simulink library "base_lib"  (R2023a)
settings: Solver=VariableStepAuto  StartTime=0.0  StopTime=10.0  RelTol=1e-3
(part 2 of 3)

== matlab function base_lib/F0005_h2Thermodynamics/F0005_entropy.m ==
function s = F0005_entropy(T,rho)
%ENTROPY
%    S = ENTROPY(T,RHO)

%    This function was generated by the Symbolic Math Toolbox version 8.7.
%    04-Nov-2021 19:06:03

t2 = rho.^2;
t3 = rho.^3;
t5 = 1.0./T;
t6 = rho./1.5508e+4;
t4 = t2.^2;
t7 = -t6;
t9 = t5.*3.3145e+1;
t10 = t6-3.9e+1./2.5e+2;
t11 = t6-6.7e+1./1.0e+2;
t12 = t6-2.17e+2./1.25e+2;
t13 = t6-7.53e+2./5.0e+2;
t14 = t6-8.31e+2./5.0e+2;
t55 = t5.*6.858999999999336e+3;
t56 = t5.*5.309999999993605e+2;
t57 = t5.*1.98899999999884e+3;
t59 = t5.*2.484000000001446e+3;
t60 = t5.*7.51000000000887e+2;
t8 = exp(t7);
t15 = t10.^2;
t16 = t11.^2;
t17 = t12.^2;
t18 = t13.^2;
t19 = t14.^2;
t20 = t9.^2.986;
t21 = t9.^5.646;
t22 = t9.^(7.91e+2./1.0e+3);
t23 = t9.^4.187;
t24 = t9.^7.249;
t25 = t9-7.164e-1;
t26 = t9-7.204e-1;
t27 = t9-1.5445;
t28 = t9-1.3444;
t29 = t9-1.4517;
t58 = -t55;
t61 = -t56;
t62 = -t57;
t63 = -t59;
t64 = -t60;
t30 = t25.^2;
t31 = t26.^2;
t32 = t27.^2;
t33 = t28.^2;
t34 = t29.^2;
t35 = t15.*(4.89e+2./1.0e+3);
t36 = t17.*(1.03e+2./1.0e+3);
t38 = t18.*(3.37e+2./2.0e+2);
t39 = t16.*2.506;
t43 = t19.*1.607;
t65 = exp(t58);
t66 = exp(t61);
t67 = exp(t62);
t68 = exp(t63);
t69 = exp(t64);
t37 = -t35;
t40 = -t36;
t41 = -t38;
t42 = -t39;
t44 = -t43;
t45 = t30.*(1.71e+2./1.0e+3);
t46 = t33.*2.245e-1;
t48 = t31.*2.785e-1;
t51 = t32.*3.967e-1;
t52 = t34.*1.304e-1;
t47 = -t45;
t49 = -t46;
t50 = -t48;
t53 = -t51;
t54 = -t52;
t70 = t37+t49;
t71 = t41+t47;
t73 = t42+t50;
t75 = t40+t54;
t78 = t44+t53;
t72 = exp(t70);
t74 = exp(t71);
t76 = exp(t73);
t77 = exp(t75);
t79 = exp(t78);
et1 = T.*4.525569467491326e-2+t4./5.78393187877481e+18-(t65.*2.518450143309456e+2)./(t65-1.0)-(t66.*2.58891537184784e+1)./(t66-1.0)+(t67.*4.75271685020088e+1)./(t67-1.0);
et2 = (t68.*(-5.68071202293286e+1))./(t68-1.0)+(t69.*9.32830592850702)./(t69-1.0)+rho.*1.0./t9.^(1.1e+1./1.0e+3).*1.345685388186742e-4+rho.*1.0./t9.^(5.11e+2./1.0e+3).*1.425437522568997e-4;
et3 = rho.*1.0./t9.^3.156e-1.*(-3.061189509930358e-4)+t2.*1.0./t9.^(1.97e+2./1.0e+3).*2.445961028609361e-9+t3.*t9.^(4.09e+2./1.0e+3).*4.94840435608013e-14;
et4 = t2.*t9.^1.444e-1.*(-6.380426347215835e-9)-rho.*t8.*t9.^(3.77e+2./5.0e+2).*8.792778927005417e-5+rho.*t9.^(9.93e+2./5.0e+2).*t79.*1.073146218725819e-5;
et5 = rho.*t9.^4.646.*t72.*8.239344544751096e-6-rho.*t9.^6.249.*t76.*1.083292654114006e-5+t3.*1.0./t9.^(2.09e+2./1.0e+3).*t77.*6.826366580922388e-15;
et6 = t3.*t8.*t9.^(3.11e+2./1.0e+3).*1.237111603428444e-13-t2.*t9.^3.187.*t74.*3.685912798034e-10;
et7 = rho.*t21.*t72.*(t5.*1.4882105e+1-6.036356e-1).*(-1.459324219757545e-6)+rho.*t24.*t76.*(t5.*1.8461765e+1-4.012628e-1).*1.494402888831571e-6;
et8 = t2.*t23.*t74.*(t5.*1.133559e+1-2.450088e-1).*8.803230948254119e-11-t3.*t22.*t77.*(t5.*8.644216-3.7860336e-1).*8.630046246425269e-15;
et9 = rho.*t20.*t79.*(t5.*2.6297243e+1-1.2254063).*(-3.593925715759608e-6)+1.888076782;
et10 = t5.*(-5.203221931700199e+2)-log(-t65+1.0).*1.0118712424e+1-log(-t66+1.0).*1.3436186752e+1;
et11 = log(-t67+1.0).*6.585061824-log(-t68+1.0).*6.302369776+log(-t69+1.0).*3.4230681224-log(t6).*8.314472;
et12 = log(t9).*(-1.2471708e+1)-t4.*t5.*4.764633820313524e-17-rho.*t9.^(4.89e+2./1.0e+3).*2.423672877126645e-3;
et13 = rho.*t9.^(9.89e+2./1.0e+3).*(-1.131310766520506e-3)+rho.*t9.^6.844e-1.*3.718903341176167e-3;
et14 = t2.*t9.^(8.03e+2./1.0e+3).*(-2.532612015624375e-8)-t3.*t9.^1.409.*2.920040416132454e-13;
et15 = t2.*t9.^1.1444.*4.635606100313556e-8+t5.*(et1+et2+et3+et4+et5+et6+et7+et8+et9).*2.7558317444e+2+rho.*t8.*t9.^(8.77e+2./5.0e+2).*4.168033876327057e-4;
et16 = t3.*t8.*t9.^1.311.*(-7.845865589306564e-13)-rho.*t21.*t72.*1.213351036409595e-5;
et17 = rho.*t20.*t79.*(-2.988159473376322e-5)+rho.*t24.*t76.*1.242517097590921e-5;
et18 = t2.*t23.*t74.*7.319421722879233e-10-t3.*t22.*t77.*7.1754277874608e-14;
et19 = 1.212238084254062e+1;
s = et10+et11+et12+et13+et14+et15+et16+et17+et18+et19;

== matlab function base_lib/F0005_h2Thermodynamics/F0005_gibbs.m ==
function g = F0005_gibbs(T,rho)
%GIBBSENERGY
%    G = GIBBSENERGY(T,RHO)

%    This function was generated by the Symbolic Math Toolbox version 8.7.
%    04-Nov-2021 19:06:06

t2 = rho.^2;
t3 = rho.^3;
t4 = 1.0./T;
t5 = rho./1.5508e+4;
t6 = -t5;
t8 = t4.*3.3145e+1;
t9 = t5-3.9e+1./2.5e+2;
t10 = t5-6.7e+1./1.0e+2;
t11 = t5-2.17e+2./1.25e+2;
t12 = t5-7.53e+2./5.0e+2;
t13 = t5-8.31e+2./5.0e+2;
t7 = exp(t6);
t14 = t9.^2;
t15 = t10.^2;
t16 = t11.^2;
t17 = t12.^2;
t18 = t13.^2;
t19 = t8.^(8.77e+2./5.0e+2);
t20 = t8.^(4.89e+2./1.0e+3);
t21 = t8.^2.986;
t22 = t8.^5.646;
t23 = t8.^(7.91e+2./1.0e+3);
t24 = t8.^(8.03e+2./1.0e+3);
t25 = t8.^(9.89e+2./1.0e+3);
t26 = t8.^1.311;
t27 = t8.^1.409;
t28 = t8.^6.844e-1;
t29 = t8.^4.187;
t30 = t8.^1.1444;
t31 = t8.^7.249;
t32 = t8-7.164e-1;
t33 = t8-7.204e-1;
t34 = t8-1.5445;
t35 = t8-1.3444;
t36 = t8-1.4517;
t37 = t32.^2;
t38 = t33.^2;
t39 = t34.^2;
t40 = t35.^2;
t41 = t36.^2;
t42 = t14.*(4.89e+2./1.0e+3);
t43 = t16.*(1.03e+2./1.0e+3);
t45 = t17.*(3.37e+2./2.0e+2);
t46 = t15.*2.506;
t50 = t18.*1.607;
t71 = rho.*t7.*t19.*5.012986845499098e-5;
t73 = t3.*t7.*t26.*9.43639666993474e-14;
t44 = -t42;
t47 = -t43;
t48 = -t45;
t49 = -t46;
t51 = -t50;
t52 = t37.*(1.71e+2./1.0e+3);
t53 = t40.*2.245e-1;
t55 = t38.*2.785e-1;
t58 = t39.*3.967e-1;
t59 = t41.*1.304e-1;
t54 = -t52;
t56 = -t53;
t57 = -t55;
t60 = -t58;
t61 = -t59;
t62 = t44+t56;
t63 = t48+t54;
t65 = t49+t57;
t67 = t47+t61;
t70 = t51+t60;
t64 = exp(t62);
t66 = exp(t63);
t68 = exp(t65);
t69 = exp(t67);
t72 = exp(t70);
et1 = t20.*4.52059+t25.*2.1101-t28.*6.93643+t71-t73+rho.*t24.*9.447562548362136e-5-rho.*t30.*1.729249419654372e-4+t3.*t4.*3.554762889834598e-13;
et2 = t7.*t19.*(-7.77414e-1)+t2.*t27.*1.633921676808176e-9+t22.*t64.*2.26312e-2+t21.*t72.*5.57346e-2-t31.*t68.*2.31752e-2;
et3 = rho.*t29.*t66.*(-2.730410110910498e-6)+t2.*t7.*t26.*4.390189186720438e-9+t2.*t23.*t69.*4.015042715686892e-10;
et4 = rho.*t31.*t68.*(rho.*3.231880319834924e-4-3.35804).*1.494402888831571e-6-rho.*t22.*t64.*(rho.*6.30642249161723e-5-1.52568e-1).*1.459324219757545e-6;
et5 = rho.*t21.*t72.*(rho.*2.072478720660304e-4-5.341668).*(-3.593925715759608e-6)+t2.*t29.*t66.*(rho.*2.17307196285788e-4-5.07522).*8.803230948254119e-11;
et6 = t3.*t23.*t69.*(rho.*1.328346659788496e-5-3.57616e-1).*(-8.630046246425269e-15);
et7 = t4.*6.258030493939e+1-t71+t73+log(-exp(t4.*(-5.309999999993605e+2))+1.0).*(2.02e+2./1.25e+2)-log(-exp(t4.*(-1.98899999999884e+3))+1.0).*(9.9e+1./1.25e+2);
et8 = log(-exp(t4.*(-6.858999999999336e+3))+1.0).*1.217+log(-exp(t4.*(-2.484000000001446e+3))+1.0).*(3.79e+2./5.0e+2)-log(-exp(t4.*(-7.51000000000887e+2))+1.0).*4.117e-1+log(t5)+log(t8).*(3.0./2.0);
et9 = rho.*t20.*2.915005158627805e-4+rho.*t25.*1.360652566417333e-4-rho.*t28.*4.472807583182873e-4+t2.*t24.*3.046028678218383e-9+t3.*t27.*3.5119974138255e-14;
et10 = t2.*t30.*(-5.575346336259904e-9)+t2.^2.*t4.*5.730530838655208e-18+t5.*(et1+et2+et3+et4+et5+et6)+rho.*t22.*t64.*1.459324219757545e-6+rho.*t21.*t72.*3.593925715759608e-6-rho.*t31.*t68.*1.494402888831571e-6;
et11 = t3.*t23.*t69.*8.630046246425269e-15-t2.*t29.*t66.*8.803230948254119e-11-4.579856474999999e-1;
g = T.*(et7+et8+et9+et10+et11).*8.314472;

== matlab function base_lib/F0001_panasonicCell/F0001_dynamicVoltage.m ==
function [dx,V] = F0001_dynamicVoltage2(in1,T,i)
%BATTERYMODEL
%    [DX,V] = BATTERYMODEL(IN1,T,I)

%    This function was generated by the Symbolic Math Toolbox version 8.7.
%    02-Apr-2022 22:29:23

x1 = in1(1,:);
x2 = in1(2,:);
x3 = in1(3,:);
x4 = in1(4,:);
x5 = in1(5,:);
t2 = abs(i);
t3 = T.^2;
t5 = T.*1.191538469793427e+2;
t4 = t2.^2;
t6 = t2.*3.727678923610498e+2;
t7 = t5+t6+1.522023870656536e+3;
t8 = 1.0./t7;
et1 = T.*1.24826954009334e-4+t2.*4.819446179569201e-3;
et2 = t3.*(-1.270473422276427e-5)-t4.*4.61451648803152e-4;
et3 = T.*t2.*7.328585354340358e-5-3.630586079057569e-2;
et4 = T.*3.12067385023335e-5+t2.*1.2048615448923e-3;
et5 = t3.*(-3.176183555691067e-6)-t4.*1.15362912200788e-4;
et6 = T.*t2.*1.83214633858509e-5-9.076465197643922e-3;
et7 = T.*1.386966155659266e-5+t2.*5.354940199521335e-4;
et8 = t3.*(-1.411637135862696e-6)-t4.*5.127240542257244e-5;
et9 = T.*t2.*8.142872615933731e-6-4.033984532286187e-3;
et10 = T.*7.801684625583374e-6+t2.*3.012153862230751e-4;
et11 = t3.*(-7.940458889227668e-7)-t4.*2.8840728050197e-5;
et12 = T.*t2.*4.580365846462724e-6-2.26911629941098e-3;
et13 = T.*4.99307816037336e-6+t2.*1.927778471827681e-4;
et14 = t3.*(-5.081893689105708e-7)-t4.*1.845806595212608e-5;
et15 = T.*t2.*2.931434141736143e-6-1.452234431623028e-3;
dx = [i+(t8.*x1)./(et1+et2+et3);i+(t8.*x2)./(et4+et5+et6);i+(t8.*x3)./(et7+et8+et9);i+(t8.*x4)./(et10+et11+et12);i+(t8.*x5)./(et13+et14+et15)];
if nargout > 1
    et16 = T.*(-3.9634064763378e-3)-t2.*3.350735047934658e-3+t3.*6.415036047911208e-5+t4.*8.829330685388394e-5+T.*t2.*7.933830899953405e-5;
    et17 = 9.538952169556378e-2;
    V = t8.*x1+t8.*x2+t8.*x3+t8.*x4+t8.*x5+i.*(et16+et17);
end

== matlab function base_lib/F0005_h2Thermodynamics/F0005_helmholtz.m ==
function a = F0005_helmholtz(T,rho)
%HELMHOLTZENERGY
%    A = HELMHOLTZENERGY(T,RHO)

%    This function was generated by the Symbolic Math Toolbox version 8.7.
%    04-Nov-2021 19:06:02

t2 = rho.^2;
t3 = rho.^3;
t4 = 1.0./T;
t5 = rho./1.5508e+4;
t6 = -t5;
t8 = t4.*3.3145e+1;
t7 = exp(t6);
et1 = t4.*6.258030493939e+1+log(-exp(t4.*(-5.309999999993605e+2))+1.0).*(2.02e+2./1.25e+2)-log(-exp(t4.*(-1.98899999999884e+3))+1.0).*(9.9e+1./1.25e+2);
et2 = log(-exp(t4.*(-6.858999999999336e+3))+1.0).*1.217+log(-exp(t4.*(-2.484000000001446e+3))+1.0).*(3.79e+2./5.0e+2)-log(-exp(t4.*(-7.51000000000887e+2))+1.0).*4.117e-1+log(t5)+log(t8).*(3.0./2.0);
et3 = rho.*t8.^(4.89e+2./1.0e+3).*2.915005158627805e-4+rho.*t8.^(9.89e+2./1.0e+3).*1.360652566417333e-4-rho.*t8.^6.844e-1.*4.472807583182873e-4+t2.^2.*t4.*5.730530838655208e-18;
et4 = t2.*t8.^(8.03e+2./1.0e+3).*3.046028678218383e-9+t3.*t8.^1.409.*3.5119974138255e-14-t2.*t8.^1.1444.*5.575346336259904e-9-rho.*t7.*t8.^(8.77e+2./5.0e+2).*5.012986845499098e-5;
et5 = t3.*t7.*t8.^1.311.*9.43639666993474e-14+rho.*t8.^5.646.*exp((t5-3.9e+1./2.5e+2).^2.*(-4.89e+2./1.0e+3)-(t8-1.3444).^2.*2.245e-1).*1.459324219757545e-6;
et6 = rho.*t8.^7.249.*exp((t5-6.7e+1./1.0e+2).^2.*(-2.506)-(t8-7.204e-1).^2.*2.785e-1).*(-1.494402888831571e-6);
et7 = rho.*t8.^2.986.*exp((t5-8.31e+2./5.0e+2).^2.*(-1.607)-(t8-1.5445).^2.*3.967e-1).*3.593925715759608e-6;
et8 = t2.*t8.^4.187.*exp((t5-7.53e+2./5.0e+2).^2.*(-3.37e+2./2.0e+2)-(t8-7.164e-1).^2.*(1.71e+2./1.0e+3)).*(-8.803230948254119e-11);
et9 = t3.*t8.^(7.91e+2./1.0e+3).*exp((t5-2.17e+2./1.25e+2).^2.*(-1.03e+2./1.0e+3)-(t8-1.4517).^2.*1.304e-1).*8.630046246425269e-15-1.4579856475;
a = T.*(et1+et2+et3+et4+et5+et6+et7+et8+et9).*8.314472;

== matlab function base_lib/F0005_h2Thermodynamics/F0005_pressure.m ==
function p = F0005_pressure(T,rho)
%PRESSURE
%    P = PRESSURE(T,RHO)

%    This function was generated by the Symbolic Math Toolbox version 8.7.
%    04-Nov-2021 19:06:02

t2 = rho.^2;
t3 = rho.^3;
t4 = 1.0./T;
t5 = rho./1.5508e+4;
t6 = -t5;
t8 = t4.*3.3145e+1;
t9 = t5-3.9e+1./2.5e+2;
t10 = t5-6.7e+1./1.0e+2;
t11 = t5-2.17e+2./1.25e+2;
t12 = t5-7.53e+2./5.0e+2;
t13 = t5-8.31e+2./5.0e+2;
t7 = exp(t6);
t14 = t9.^2;
t15 = t10.^2;
t16 = t11.^2;
t17 = t12.^2;
t18 = t13.^2;
t19 = t8.^(8.77e+2./5.0e+2);
t20 = t8.^2.986;
t21 = t8.^5.646;
t22 = t8.^(7.91e+2./1.0e+3);
t23 = t8.^1.311;
t24 = t8.^4.187;
t25 = t8.^7.249;
t26 = t8-7.164e-1;
t27 = t8-7.204e-1;
t28 = t8-1.5445;
t29 = t8-1.3444;
t30 = t8-1.4517;
t31 = t26.^2;
t32 = t27.^2;
t33 = t28.^2;
t34 = t29.^2;
t35 = t30.^2;
t36 = t14.*(4.89e+2./1.0e+3);
t37 = t16.*(1.03e+2./1.0e+3);
t39 = t17.*(3.37e+2./2.0e+2);
t40 = t15.*2.506;
t44 = t18.*1.607;
t38 = -t36;
t41 = -t37;
t42 = -t39;
t43 = -t40;
t45 = -t44;
t46 = t31.*(1.71e+2./1.0e+3);
t47 = t34.*2.245e-1;
t49 = t32.*2.785e-1;
t52 = t33.*3.967e-1;
t53 = t35.*1.304e-1;
t48 = -t46;
t50 = -t47;
t51 = -t49;
t54 = -t52;
t55 = -t53;
t56 = t38+t50;
t57 = t42+t48;
t59 = t43+t51;
t61 = t41+t55;
t64 = t45+t54;
t58 = exp(t56);
t60 = exp(t57);
t62 = exp(t59);
t63 = exp(t61);
t65 = exp(t64);
et1 = t3.*t4.*3.554762889834598e-13-t7.*t19.*7.77414e-1+t21.*t58.*2.26312e-2+t20.*t65.*5.57346e-2-t25.*t62.*2.31752e-2;
et2 = rho.*t8.^(8.03e+2./1.0e+3).*9.447562548362136e-5-rho.*t8.^1.1444.*1.729249419654372e-4+t2.*t8.^1.409.*1.633921676808176e-9+t8.^(4.89e+2./1.0e+3).*4.52059;
et3 = t8.^(9.89e+2./1.0e+3).*2.1101-t8.^6.844e-1.*6.93643+rho.*t7.*t19.*5.012986845499098e-5-rho.*t24.*t60.*2.730410110910498e-6+t2.*t7.*t23.*4.390189186720438e-9;
et4 = t3.*t7.*t23.*(-9.43639666993474e-14)+t2.*t22.*t63.*4.015042715686892e-10+rho.*t25.*t62.*(rho.*3.231880319834924e-4-3.35804).*1.494402888831571e-6;
et5 = rho.*t21.*t58.*(rho.*6.30642249161723e-5-1.52568e-1).*(-1.459324219757545e-6)-rho.*t20.*t65.*(rho.*2.072478720660304e-4-5.341668).*3.593925715759608e-6;
et6 = t2.*t24.*t60.*(rho.*2.17307196285788e-4-5.07522).*8.803230948254119e-11-t3.*t22.*t63.*(rho.*1.328346659788496e-5-3.57616e-1).*8.630046246425269e-15;
p = T.*rho.*(t5.*(et1+et2+et3+et4+et5+et6)+1.0).*8.314472;

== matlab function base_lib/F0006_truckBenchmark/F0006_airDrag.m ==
function Fa = F0006_airDrag(v, par)
% inputs:
% v [m/s] - vehicle speed

% parameters:
rho_air = par.rho_air;
A_f     = par.A_f; % 10;
C_d     = par.C_d; % 0.5;

% output:
Fa = 1/2 * rho_air .* A_f .* C_d .* v.^2;
end

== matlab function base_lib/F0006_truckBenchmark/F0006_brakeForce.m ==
function Fb = F0006_brakeForce(brake, par)
% inputs:
% brake [0,1] - brake signal

% parameters:
m    = par.m;
g    = 9.82;
gain = par.gain;

% output
Fb = min(min(max(brake,0),1) .* gain, m.*g);
end

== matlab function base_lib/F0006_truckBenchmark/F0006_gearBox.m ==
function [Tq_out, w_in] = F0006_gearBox(Tq_in, w_out, gear_ratio, par)
% parameters
fd_ratio = par.fd_ratio;
eta_gb   = par.eta_gb;

% combined drive ratio
gam = fd_ratio .* gear_ratio;

% torque on wheel
Tq_out = Tq_in .* gam .* eta_gb.^(sign(Tq_in));

% electric motor angular speed
w_in = w_out .* fd_ratio .* gear_ratio;

end

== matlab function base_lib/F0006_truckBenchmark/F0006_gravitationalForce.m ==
function Fg = F0006_gravitationalForce(alpha, par)
% inputs:
% alpha [rad] - road slope

% parameters:
m       = par.m;
g       = 9.82;

% output
Fg =   m .* g .* sin(alpha);
end

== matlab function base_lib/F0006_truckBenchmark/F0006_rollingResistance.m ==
function Fr = F0006_rollingResistance(v, alpha, par)
% inputs:
% v     [m/s] - vehicle speed
% alpha [rad] - road slope

% parameters:
c_r0 = par.c_r0;
c_r1 = par.c_r1;
m    = par.m;
g    = 9.82;

% m/s -> km/h
v_k = v * 3.6;

% rolling resistance coefficient
c_r = c_r0 + c_r1 .* v_k.^2;

% output
Fr =  c_r .* m .* g .* cos(alpha);
end

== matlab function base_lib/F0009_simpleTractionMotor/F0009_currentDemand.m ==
function [Q_gen, I_em] = F0009_currentDemand(Tq_em, V, w_em, par)

% Parameters
e     = par.e;
c1    = par.c1;
c2    = par.c2;
c3    = par.c3;

P_0 = c1 + c2 * w_em + c3 * w_em.^2;
P_em = Tq_em .* w_em;
P_tot = P_em + P_0;

% Motor power
P_el  = 1/e*P_tot;
I_m   = P_el ./ V;

% Generator power
P_el  = e*P_tot;
I_g   = P_el ./ V;

% switching variables
ym = (tanh(P_tot - pi) + 1)/2;
yg = (tanh(pi - P_tot) + 1)/2;

% Current
I_em = ym .* I_m + yg .* I_g;

% Power loss
Q_gen = abs(abs(I_em) .* V - abs(Tq_em .* w_em));

end

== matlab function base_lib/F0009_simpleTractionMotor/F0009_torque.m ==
function Tq_em = F0009_torque(V, I, w, par)

% Output size
Tq_em = 0;

% Parameters
e     = par.e;
c1    = par.c1;
c2    = par.c2;
c3    = par.c3;

% minimum speed
w   = max(w, 10);

% power loss
P_0 = c1 + c2 * w + c3 * w.^2;

% Input power
P = V .* I;

% Motor power & torque
P_m  = (e * P - P_0);
Tq_m = P_m ./ w; 

% Generator power & torque
P_g  = P./e + P_0;
Tq_g = P_g ./ w;

% output depending on motor/generator mode
if I > 0
    Tq_em = Tq_m;
else
    Tq_em = Tq_g;
end

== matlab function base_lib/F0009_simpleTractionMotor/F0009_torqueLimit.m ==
function Tq_em = F0009_torqueLimit(Tq_req, V, w_em, par)

% Parameters
I_max = par.I_max;
e     = par.e;
c1    = par.c1;
c2    = par.c2;
c3    = par.c3;

% Losses
P_0 = c1 + c2 * w_em + c3 * w_em.^2 ;

% Traction
P_1_trac = I_max .* V;         
P_2_trac = (P_1_trac - P_0)/e;
Tq_trac  = P_2_trac ./ w_em;  % maximum traction torque

% Recuperation
P_1_recup = I_max .* V;
P_2_recup = e.*P_1_recup + P_0;
Tq_recup  = -P_2_recup ./ w_em ;  % minimum recuperation torque

% limit
Tq_em = Tq_req;
Tq_em( Tq_em > Tq_trac)  = Tq_trac;
Tq_em( Tq_em < Tq_recup) = Tq_recup;

end

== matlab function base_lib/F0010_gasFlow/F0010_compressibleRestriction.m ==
function W = F0010_compressibleRestriction(p_us, p_ds, T_us, cp_m, R_m, A_t, par)
W = 0;

% parameters
C_d    = par.C_d;        % [?]      - discharge coefficient

Pi_lin = par.Pi_lin;

% Ratio of specific heats
g = cp_m/(cp_m - R_m);

% Pressure ratio
pr = p_ds ./ p_us;

% Flow
pr_crit = (2/(1+g)).^( g/(g-1) );
Pi      = max(pr, pr_crit);
Pi      = min(Pi,1);
Phi     = sqrt( 2*g./(g-1) .* ( Pi.^(2/g) - Pi.^((g+1)/g)) );
Phi_lin = sqrt( 2*g./(g-1) .* ( Pi_lin.^(2/g) - Pi_lin.^((g+1)/g)) );
Phi(Pi > Pi_lin) = Phi_lin .* (1-Pi)./(1-Pi_lin);
W       = p_us ./ sqrt(R_m.*T_us) .* A_t .* C_d .* Phi;

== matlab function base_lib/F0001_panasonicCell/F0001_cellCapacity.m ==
function Q0 = F0001_cellCapacity(T)
% Fit to cycle data from
% Li-Ion Battery Model Performance for Automotive Drive
% Cycles with Current Pulse and EIS Parameterization
% Kolmeyer et al, 
% 978-1-5090-3953-1/$31.00 ©2017 IEEE

% parameters
a0 = 2.5718;
a1 = 0.0307;
a2 = -0.0006;

Q0 = a0 + a1.*T + a2 .*T^2;
end

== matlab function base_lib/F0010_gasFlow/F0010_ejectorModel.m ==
function [W_p, W_s, phi, w] = F0010_ejectorModel(P_p, P_s, P_b, T_p, p_sat, RH_s, par)

% determine output sizes
W_p = 0;
W_s = 0;
phi = 0;
w   = 0;

% parameters
C_d    = par.C_d;        % [-]   - Discharge coefficient
D_t    = par.D_t;        % [m]   - Nozzle throat diameter
A_t    = pi*(D_t/2)^2;   % [m2]  - Nozzle throat area
c_0    = par.c_0;
c_1    = par.c_1;
Pi_lin = par.Pi_lin;

% gas properties
M_H2  = 2.016e-3;        % [kg/mol] - hydrogen gas molecular weight
M_H2O = 36.030e-3;       % [kg/mol] - water molecular weight
R_g   = 8.314 / M_H2;    % [J/kg*K] - hydrogen gas constant 
cp    = 14.31e3;         % [J/kg*K] - hydrogen gas specific heat @ 300 K
g     = cp/(cp - R_g);     % [-]      - ratio of specific heats

% pressure ratio
pr = P_b ./ P_p;

% primary flow
pr_crit = (2/(1+g)).^( g/(g-1) );
Pi      = max(pr, pr_crit);
Pi      = min(Pi,1);
Phi     = sqrt( 2*g./(g-1) .* ( Pi.^(2/g) - Pi.^((g+1)/g)) );
Phi_lin = sqrt( 2*g./(g-1) .* ( Pi_lin.^(2/g) - Pi_lin.^((g+1)/g)) );
Phi(Pi > Pi_lin) = Phi_lin .* (1-Pi)./(1-Pi_lin);
W_p     = P_p ./ sqrt(R_g.*T_p) .* A_t .* C_d .* Phi;


% recirculation ratio
t   = ((tanh( (pr - pr_crit)*20 ) ) + 1)/2;
phi = (c_0 + c_1.*pr) .* (1-t); 

% secondary flow
x_H2O   = p_sat .* RH_s ./ P_s;
y_H2O   = M_H2O .* x_H2O ./ (M_H2O .* x_H2O + M_H2.*(1 - x_H2O));
W_s     = phi .* W_p ./ (1 - y_H2O);

% entrainment
w = W_s ./ W_p;

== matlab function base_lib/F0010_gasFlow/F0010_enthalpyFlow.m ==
function H = F0010_enthalpyFlow(W, T_1, T_2, par)
% parameters
cp_j = par.cp_j; % [J/kgK]  - Specific heats

% Upstream & downstream total pressure
% Switch variable
y = (tanh(W*1e4-pi) + 1)/2;

% Upstream temperature
T_us =  y.*T_1 + (1-y).*T_2;

% Enthalpy flow
H = W .* T_us .* cp_j;
end

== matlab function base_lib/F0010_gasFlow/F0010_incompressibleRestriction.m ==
function W = F0010_incompressibleRestriction(p_1, T_1,  p_2, T_2, par)
% output size
W = zeros(4,1);

% parameters
C_d = par.C_d;   % [?]      - Convective flow coefficient
D_t = par.D_t;        % [m]   - Nozzle throat diameter
A_t = pi*(D_t/2)^2;   % [m2]  - Nozzle throat area
M_j = par.M_j; % [kg/mol] - Molar masses
R_j = par.R_j; % [J/kgK]  - Specific gas constants

% Upstream & downstream total pressure
p_1_tot  = sum(p_1);
p_2_tot  = sum(p_2);

% Pressure & temperature drop
dp = p_1_tot - p_2_tot;

dp_tan = dp.*par.tan_par;

% Switch variable
y = (tanh(dp_tan) + 1)/2;

% Upstream pressure, temperature & concentration
p_us = y.*p_1 + (1-y).*p_2;
T_us = y.*T_1 + (1-y).*T_2;

% Upstream total pressure
p_tot = sum(p_us);

% Upstream mole fractions
x_us = p_us ./ p_tot;

% Average molar mass
M_avg = sum(x_us .* M_j);

% Mole fraction to mass fraction
w_us = x_us .* M_j ./ M_avg;

% mixture gas constant
R_m = sum(w_us .* R_j);

% Total mass flow
W_c = C_d .* A_t .* sqrt(p_tot./(R_m.*T_us)).*sqrt(abs(dp));
W_c = tanh(dp_tan) .* W_c;

% linear region
dp_lin  = par.dp_lin;
W_c_lin = C_d .* A_t .* sqrt(p_tot./(R_m.*T_us)) .* abs(dp) ./ sqrt(dp_lin);
W_c(abs(dp) < dp_lin) = tanh(dp_tan) .* W_c_lin;

% Distribute mass flow accoring to mass ratios
W   = W_c .* w_us;
end

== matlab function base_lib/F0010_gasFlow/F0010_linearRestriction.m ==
function W = F0010_linearRestriction(p_us,  p_ds,  par)
% parameters
C_d = par.C_d;   % [?]    - Convective flow coefficient

% Pressure & temperature drop
dp = p_us - p_ds;

% linear flow
W = C_d .* max(dp,0) ;

end

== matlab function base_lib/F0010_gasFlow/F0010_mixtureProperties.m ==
function [x, cp_m, cv_m, R_m] = F0010_mixtureProperties(p, par)
% Parameters
cp_j = par.cp_j; % [J/kgK]  - Specific heats
M_j  = par.M_j;  % [kg/mol] - Molar masses
R_j  = par.R_j;  % [J/kgK]  - Specific gas constant

% Mole fractions
p_tot = sum(p);
x     = p ./ p_tot;

% Average molar mass
M_avg = sum(x .* M_j);

% Mole fraction to mass fraction
w = x .* M_j ./ M_avg;

% Mixture gas constant
R_m = sum(w .* R_j);

% Mixture specific heats
cp_m = sum(w .* cp_j);
cv_m = cp_m - R_m;

end

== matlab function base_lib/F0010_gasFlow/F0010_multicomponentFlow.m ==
function W_split = F0010_multicomponentFlow(p_us, W_tot, par)
% Parameters
cp_j = par.cp_j; % [J/kgK]  - Specific heats
M_j  = par.M_j;  % [kg/mol] - Molar masses
R_j  = par.R_j;  % [J/kgK]  - Specific gas constant

% Mole fractions
p_tot = sum(p_us);
x     = p_us ./ p_tot;

% Average molar mass
M_avg = sum(x .* M_j);

% Mole fraction to mass fraction
w = x .* M_j ./ M_avg;

% outlet species convective mass flow
W_split = W_tot .* w;

end

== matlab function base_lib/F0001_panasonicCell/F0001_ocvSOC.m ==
% A Generalized SOC-OCV Model for Lithium-Ion
% Batteries and the SOC Estimation for LNMCO Battery
% Zhang et al, Energies
% doi:10.3390/en9110900

% Fit to OCV-data from
% Li-Ion Battery Model Performance for Automotive Drive
% Cycles with Current Pulse and EIS Parameterization
% Kolmeyer et al, 
% 978-1-5090-3953-1/$31.00 ©2017 IEEE

function U = F0001_ocvSOC(SOC)
% inputs x [-] - state of charge

% parameters
a =  2.0966;
b = -0.0055;
c = -0.2433;
d =  2.3054;
m =  3.0965;
n =  0.6010;

% OCV
x = SOC;
U = a + b * (-log(x)).^m + c .* x + d.*exp( n.*(x-1));
end

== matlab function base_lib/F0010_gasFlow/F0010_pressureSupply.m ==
function p_out = F0010_pressureSupply(p_tot, x_H2_dry, x_O2_dry, RH, p_sat, par)

% mole fraction of vapor
x_H2O = RH .* p_sat ./ p_tot;

% mole fraction hydrogen
x_H2 = (1-x_H2O).*x_H2_dry;

% mole fraction hydrogen
x_O2 = (1-x_H2O).*x_O2_dry;

% mole fraction nitrogen
x_N2 = 1 - x_H2 - x_O2 - x_H2O;




% partial pressures
p_out = [x_H2; x_O2; x_H2O; x_N2] .* p_tot;

end

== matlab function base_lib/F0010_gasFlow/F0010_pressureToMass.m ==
function m = F0010_pressureToMass(p, T, par)
% parameters
Rj     = par.R_j;
V      = par.V;

% mass
m = p .* V ./ (Rj .* T);
end

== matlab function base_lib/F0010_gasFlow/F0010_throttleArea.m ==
function A_t = F0010_throttleArea(alpha, par)
% model parameters
a0 = par.a0;
a1 = par.a1;
a2 = par.a2;

% effective area
A_t = a0 + a1.*alpha + a2 .* alpha.^2;
end

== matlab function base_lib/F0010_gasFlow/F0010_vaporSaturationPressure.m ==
function p_sat = F0010_vaporSaturationPressure(T)
% Journal of Physical and Chemical Reference Data 31,
% 387 (2002); https://doi.org/10.1063/1.1461829
c1 =  -7.85951783;
c2 =   1.84408259;
c3 = -11.7866497;
c4 =  22.6807411;
c5 = -15.9618719;
c6 =   1.80122502;

% critical temperature & pressure
Tcrit = 647.096;
pcrit = 22.06e6;

% saturation pressure as function of temperature
p_sat = pcrit*exp(Tcrit./T .* ( ...
    c1*(1-T./Tcrit) + ...
    c2*(1-T./Tcrit).^1.5 + ...
    c3*(1-T./Tcrit).^3 + ...
    c4*(1-T./Tcrit).^3.5 + ...
    c5*(1-T./Tcrit).^4 + ...
    c6*(1-T./Tcrit).^7.5 ));

p_sat = real(p_sat);
end

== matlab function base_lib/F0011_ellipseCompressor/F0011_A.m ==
function A = F0011_A(N_corr_n, par)
% parameters
u1 = N_corr_n;
u2 = par.C_a(1);
u3 = par.C_a(2);
u4 = par.C_a(3);
u5 = par.Delta_h_max;
u6 = par.Wc_max_map;

% output
A = -( u5./u6 ).*( u2.*u1 ./( (1 + u3.*u1.^2).^u4 ));
end

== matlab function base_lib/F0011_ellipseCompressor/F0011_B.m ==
function B = F0011_B(N_corr_n, par)
% parameters
u1 = N_corr_n;
u2 = par.C_b(1);
u3 = par.C_b(2);
u4 = par.Delta_h_max;

% output
B = u4 .* ( u2 .* u1.^2 + u3 .* u1^3 );
end

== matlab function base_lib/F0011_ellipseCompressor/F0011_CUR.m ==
function CUR = F0011_CUR(N_corr_n, par)
% parameters
a1     = par.C_cur(1);
a2     = par.C_cur(2);
a3     = par.C_cur(3);

% Speed ratio
N = N_corr_n;

% output
CUR = a1 + a2.*N.^a3;
end

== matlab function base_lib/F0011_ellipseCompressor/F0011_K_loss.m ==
function K_loss = F0011_K_loss(W_corr, N_corr, par)
% parameters
rho1   = par.rho1;
D      = par.D_2;
C_loss = par.C_loss;

% output
K_loss = 1 + C_loss .* ( rho1.*D.^3 .* pi/60 ) .* (N_corr./W_corr);
end

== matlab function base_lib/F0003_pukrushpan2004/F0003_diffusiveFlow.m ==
function W = F0003_diffusiveFlow(lambda_an, lambda_m, lambda_ca, T, par)

% parameters
A   = par.A_fc; % [cm2] - cell area
t_m = par.t_m;  % [cm]  - membrane thickness

% constants
F     = 96485;  % [C/mol]   - Faradays constant
R     = 8.314;  % [J/(molK] - gas constant 
M_H2O = 0.018;  % [kg/mol]  - water molecular mass

rho_mb_dry = 0.002; % [kg/cm^3] - membrane dry density;
M_mb_dry   = 1.1;   % [kg/mol]  - membrane dry equivalent weight 

% membrane diffusivity
D                  = 1e-6;
D(lambda_m >= 2)   = 1e-6 * (1 + 2*(lambda_m-2));
D(lambda_m >= 3)   = 1e-6 * (3 - 1.67*(lambda_m-3));
D(lambda_m >= 4.5) = 1.25e-6;
D_w                = 12 * D.*exp(2416*(1/303 - 1/T));

% Water concentrations on each side
c_an = rho_mb_dry ./ M_mb_dry .* lambda_an; % [mol/cm3] - water concentration at anode
c_ca = rho_mb_dry ./ M_mb_dry .* lambda_ca; % [mol/cm3] - water concentration at cathode

% Diffusive flow
W = M_H2O .* A .* D_w .* (c_an - c_ca)/t_m;

end

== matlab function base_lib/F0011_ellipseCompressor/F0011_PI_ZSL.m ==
function PI_ZSL = F0011_PI_ZSL(N_corr_n, par)
% parameters
PI_max = par.PI_max_map;
a1     = par.C_PIzs(1);
a2     = par.C_PIzs(2);

% Speed ratio
N = N_corr_n;

% output
PI_ZSL  = 1 + (PI_max - 1) .* ( a1.*N.^a2 );
end

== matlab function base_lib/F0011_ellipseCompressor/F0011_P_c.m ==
function P_c = F0011_P_c(W_c, T_us, T_ds, par)
% parameters
cp  = par.Cp_air;

% compressor work
P_c = cp .* W_c .* (T_ds - T_us);
end

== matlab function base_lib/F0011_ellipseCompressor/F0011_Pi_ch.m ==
function Pi_ch = F0011_Pi_ch(N_corr_n, par)
% parameters
PI_max = par.PI_max_map;
a1     = par.C_PIch(1);
a2     = par.C_PIch(2);
a3     = par.C_PIch(3);

% Speed ratio
N = N_corr_n;

% output
Pi_ch  = PI_max .* ( a1 + a2.*N.^a3 );
end

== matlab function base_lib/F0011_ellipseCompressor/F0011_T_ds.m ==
function T_ds = F0011_T_ds(Pi_c, T_us, eta_c, par)
% model constants
g = par.gamma_air;

% compressor out temperature (adiabatic)
T_ds = T_us + T_us ./ eta_c .* ( Pi_c.^((g-1)/g)  - 1  );
end

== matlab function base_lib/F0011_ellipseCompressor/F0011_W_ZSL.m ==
function W_ZSL = F0011_W_ZSL(N_corr_n, par)
% parameters
Wc_max = par.Wc_max_map;
a1     = par.C_Wzs(1);
a2     = par.C_Wzs(2);

% Speed ratio
N = N_corr_n;

% output
W_ZSL = Wc_max .* a1 .* N.^a2;
end

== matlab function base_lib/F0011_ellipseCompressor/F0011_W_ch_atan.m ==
function W_ch_atan = F0011_W_ch_atan(N_corr_n, par)
% parameters
Wc_max = par.Wc_max_map;
a1     = par.C_Wch(1);
a2     = par.C_Wch(2);
a3     = par.C_Wch(3);
a4     = par.C_Wch(4);

% Speed ratio
N = N_corr_n;

% output
W_ch_atan = Wc_max .* (a1 + a2 .* atan( a3.*N - a4));
end

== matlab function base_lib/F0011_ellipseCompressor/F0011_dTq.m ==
function dw_c = F0011_dTq(Tq_em, Tq_c, w_c, par)
% parameters
J_c = par.J_c;
c   = par.c_fric;

% shaft friction
Mf = c .* w_c;

% turbo shaft dynamics
% Model 8.3
dw_c = 1/J_c .* ( Tq_em - Tq_c - Mf);

end

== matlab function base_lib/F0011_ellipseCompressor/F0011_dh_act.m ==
function dh_act = F0011_dh_act(W_c_corr, K_loss, B, A)
% inputs
u1 = W_c_corr;
u2 = K_loss;
u3 = B;
u4 = A;

% actual enthalpy change
dh_act = u2 .* ( u3 + u4 .* u1 );
end

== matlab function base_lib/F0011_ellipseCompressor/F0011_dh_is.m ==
function dh_is = F0011_dh_is(Pi_c, par)
% inputs
u1 = Pi_c;

% parameters
cp_air = par.Cp_air;
T_ref  = par.T_ref;
g      = par.gamma_air;

% isentropic enthalpy change
dh_is = cp_air .* T_ref .* ( u1.^((g - 1)./g) - 1 );
end

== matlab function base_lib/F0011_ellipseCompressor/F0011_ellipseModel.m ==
function W_corr = F0011_ellipseModel(Pi_c, Pi_ch, PI_ZSL, CUR, W_ZSL, W_ch, par)
% inputs
u1 = min(Pi_c, PI_ZSL);
u2 = Pi_ch;
u3 = PI_ZSL;
u4 = CUR;
u5 = W_ZSL;
u6 = W_ch;


% inputs
u1 = min(Pi_c, PI_ZSL);
u2 = Pi_ch;
u3 = PI_ZSL;
u4 = CUR;
u5 = W_ZSL;
u6 = W_ch;

% Surge / Regular / Choke
if (Pi_c >  PI_ZSL)
    W_corr = W_ZSL - (Pi_c - PI_ZSL)./par.alpha_kPiW0;
elseif (Pi_c < Pi_ch)
    W_corr = W_ch;
else
    W_corr = u5 + (u6-u5).*( (1 - ( (u1-u2)./(u3-u2) ).^u4).^(1./u4) );
end

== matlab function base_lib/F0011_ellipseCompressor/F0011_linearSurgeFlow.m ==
function W_corr_surge = F0011_linearSurgeFlow(W_ZSL, Pi_ZSL, Pi_c, par)
% Surge flow
W_corr_surge = W_ZSL - (Pi_c - Pi_ZSL)./par.alpha_kPiW0;

% Saturation
W_corr_surge(W_corr_surge < 1e-4) = 1e-4;
end

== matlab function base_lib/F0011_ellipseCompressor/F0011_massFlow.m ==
function W_c = F0011_massFlow(p_1, p_2, T_1, w_c, par)
% pressure ratio
Pi_c = p_2 ./ p_1;

% speed correction
[~, N_corr_n] = F0011_speedCorrection(w_c, T_1, par);

% base functions
Pi_ch  = F0011_Pi_ch(N_corr_n, par);
PI_ZSL = F0011_PI_ZSL(N_corr_n, par);
CUR    = F0011_CUR(N_corr_n, par);
W_ZSL  = F0011_W_ZSL(N_corr_n, par);
W_ch   = F0011_W_ch_atan(N_corr_n, par);

% corrected flow
W_corr = F0011_ellipseModel(Pi_c, Pi_ch, PI_ZSL, CUR, W_ZSL, W_ch, par);

% Uncorrect
W_c = W_corr .* (p_1./par.p_ref) ./ sqrt( T_1./par.T_ref);

end

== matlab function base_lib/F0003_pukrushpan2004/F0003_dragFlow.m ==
function W = F0003_dragFlow(I, lambda)

% parameters
F          = 96485;  % [C/mol]   - Faradays constant
M_H2O      = 0.018;  % [kg/mol]  - water molecular mass

% electro-osmotic drag coefficient
n_d = 0.0029 .* lambda.^2 + 0.05 .* lambda;

% Drag flow
W =  M_H2O .* n_d .* I / F;
end

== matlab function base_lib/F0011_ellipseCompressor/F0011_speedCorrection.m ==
function [N_corr, N_corr_n] = F0011_speedCorrection(w_c, T, par)
% rad/sec -> rpm
N = w_c .* 30/pi;

% speed correction
N_corr = N ./sqrt(T./par.T_ref);

% speed ratio
N_corr_n = N_corr ./ par.Nc_max_map;
end

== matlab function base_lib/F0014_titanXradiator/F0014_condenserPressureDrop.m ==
function dp = F0014_condenserPressureDrop(T, p, W, par)

% parameters
StS  = par.StS;
HtH  = par.HtH;
R    = par.R_air;
c_dp = par.c_dp; 

% Area
A = StS .* HtH;

% Velocity
v = W .* R .* T ./ (p.*A);

% pressure drop
dp = c_dp(1) .* v.^2 + c_dp(2) .* v;

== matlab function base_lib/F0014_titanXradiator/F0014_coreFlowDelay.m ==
function t = F0014_coreFlowDelay(W, par)

% parameters
rho = par.rho_clt;
HtH = par.HtH;
StS = par.StS;
CdT = par.CdT;

% approximate core inner flow area
A = 0.15 .* CdT .* StS;

% flow velocity
v = max(W ./ ( rho .* A), 0.01);

% time delay
t = min(HtH ./ v, 20);

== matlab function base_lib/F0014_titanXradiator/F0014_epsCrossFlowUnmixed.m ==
function e = F0014_epsCrossFlowUnmixed(NTU, C)
N = NTU;

N = max(N, 0);

n = N.^(-0.22);

% tanhyp switch for C approaching zero
y = (tanh(C*1e2 - pi) + 1 )./2;

% Holman, Table 10.3, Cross flow, both fluids unmixed:
e1  = 1 - exp( ( exp( -N.*C.*n ) - 1 )./(C.*n) );

% C = 0
e0 = 1 - exp(-N);

% output
e = y.*e1 + (1-y).*e0;

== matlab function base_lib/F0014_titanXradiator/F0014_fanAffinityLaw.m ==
function [q1, dp1, P1] = F0014_fanAffinityLaw(n1, q2, par)
% Source:
% https://www.engineeringtoolbox.com/fan-affinity-laws-d_196.html

% parameters
dp2 = par.dp2;
P2  = par.P2;
n2  = par.n2;
d1  = par.d1;
d2  = par.d2;

% Affinity laws
q1  = q2  .* (n1./n2)    .* (d1./d2).^3;
dp1 = dp2 .* (n1./n2).^2 .* (d1./d2).^2;
P1  = P2  .* (n1./n2).^3 .* (d1./d2).^5;

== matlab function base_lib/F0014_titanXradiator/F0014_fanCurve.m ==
function dp = F0014_fanCurve(q, dp0_n, par)

% parameters
dpr = par.dpr;
dp0 = par.dp0;
q0  = par.q0;

% pressure drop/increase
temp = (q ./ q0).^2;
dp   = max(dpr .* temp, dp0_n - dp0 .* temp);

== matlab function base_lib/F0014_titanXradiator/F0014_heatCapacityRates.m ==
function [C_min, C_max, C_air, C_clt] = F0014_heatCapacityRates(W_air, W_cl, par)

% parameters
cp_air = par.cp_air;
cp_clt = par.cp_clt;

% heat capacity rates
C_air = W_air.*cp_air;
C_clt = W_cl.*cp_clt;

% max/min rates
C_min = min(C_air, C_clt);
C_max = max(C_air, C_clt);

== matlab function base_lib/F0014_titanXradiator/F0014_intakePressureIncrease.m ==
function dp = F0014_intakePressureIncrease(T, p, v, par)

% parameters
zeta = par.zeta;
R    = par.R_air;

% density
rho = p ./ (R.*T);

% pressure drop
dp = 1/2 .* zeta .* rho .* v.^2;

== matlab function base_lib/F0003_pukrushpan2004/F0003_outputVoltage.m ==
function [V, Q_gen] = F0003_outputVoltage(I, p_an, p_ca, p_sat, lambda_m, T, par)
% ref: Control-Oriented Modeling and Analysis for Automotive Fuel Cell Systems
% authors: Jay T. Pukrushpan, Huei Peng, Anna G. Stefanopoulou
% J. Dyn. Sys., Meas., Control. Mar 2004
% https://doi.org/10.1115/1.1648308

% specify output sizes
Q_gen = 0;
V     = 0;

% parameters
A = par.A_fc; % [cm2]       - cell area
j = I ./ A;

% partial pressures
p_H2     = p_an(1); % [Pa] - hydrogen partial pressure
% p_H2O_an = p_an(2); % [Pa] - water --
% p_N2_an  = p_an(3); % [Pa] - nitrogen --
p_O2     = p_ca(2); % [Pa] - oxygen --
p_H2O_ca = p_ca(3); % [Pa] - water --
p_N2_ca  = p_ca(4); % [Pa] - nitrogen --

% parameters
c1 = 10;

% constants
R     = 8.314;     % [J/(K mol)] - Gas constant
F     = 96485;     % [C/mol]     - Faradays constant
n     = 2;         % [-]         - moles of electrons transfered per mole hydrogen reacted
E0    = 1.229;     % [V]         - standard potential
P_atm = 1.01325e5; % [Pa]        - atm. pressure
p0    = 1e5;       % [Pa]        - std. pressure
dh    = 285.8e3;   % [J/mol]     - heat of formation (liquid)
% dh    = 241.8e3;   % [J/mol]     - heat of formation (vapor)

% total pressures
% P_an = p_H2 + p_H2O_an + p_N2_an;
P_ca = p_O2 + p_H2O_ca + p_N2_ca;

% reversible voltage
E = E0 - 8.5e-4 .* (T-298.15) + R*T/(n*F) * log(p_H2./p0 .* sqrt( max(p_O2./p0,0) ));

% activation overvoltage
v0 = 0.279 - 8.5e-4 .* (T - 298.15) + 4.3085e-5 .* T .* (log((P_ca/P_atm - p_sat./P_atm)/1.01325) + 1/2 * log(0.1173*(P_ca/P_atm - p_sat./P_atm)/1.01325));
va = (-1.618e-5 * T + 1.618e-2) .* ( p_O2./P_atm./0.1173 + p_sat./P_atm ).^2 + (1.8e-4 * T - 0.166).*(p_O2./ P_atm/0.1173 + p_sat./P_atm) + (-5.8e-4 * T + 0.5736);
V_act = v0 + va.*(1 - exp(-c1.*j));

% ohmic overvoltage
b11     = 0.005139;
b12     = 0.00326;
b2      = 350;
t_m     = 0.01275;
sigma_m = (b11 .* max(lambda_m,1) - b12) .* exp( b2 .*( 1./303 - 1./T ) );
R_ohm   = t_m ./ sigma_m;
V_ohm   = j .* R_ohm;

% concentration overvoltage
temp         = (p_O2./P_atm./0.1173 + p_sat./P_atm);
c2           = (8.66e-5 .* T - 0.068) .* temp + ( -1.60e-4 * T + 0.54);
c2(temp < 2) = (7.16e-4 .* T - 0.622) .* temp + ( -1.45e-3 * T + 1.68);
c3           = 2;
j_max        = 2.2;
V_con        = j .* (c2 .* j/j_max).^c3;

% Output voltage
V = E  - V_act - V_ohm - V_con;

% Heat generation
P_elec = j.*A .* V;              % [W] - electric power
P_tot  = j .*A ./ (2*F) .* dh;   % [W] - total power
Q_gen  = P_tot - P_elec;         % [W] - heat generation

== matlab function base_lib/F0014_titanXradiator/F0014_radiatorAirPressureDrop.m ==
function dp = F0014_radiatorAirPressureDrop(v, par)
% parameters
CdT   = par.CdT;
c_dp  = par.c_dp_air;
rho   = par.rho_air;

% pressure drop
dp = CdT .* rho .* ( c_dp(1) .* v.^2 + c_dp(2) .* v );

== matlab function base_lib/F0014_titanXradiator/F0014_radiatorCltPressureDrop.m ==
function dp = F0014_radiatorCltPressureDrop(v, par)
% parameters
HtH   = par.HtH;
c_dp  = par.c_dp_clt;
rho   = par.rho_clt;

% pressure drop
dp = HtH .* rho .* ( c_dp(1) .* v.^2 + c_dp(2) .* v );

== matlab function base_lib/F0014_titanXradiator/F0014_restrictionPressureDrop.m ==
function dp = F0014_restrictionPressureDrop(T,p,W,par)

% parameters
zeta = par.zeta;
R    = par.R_air;
A    = par.A;

% density
rho = p ./ (R.*T);

% velocity
v = W ./ (rho.*A);

% pressure drop
dp = 1/2 .* zeta .* rho .* v.^2;

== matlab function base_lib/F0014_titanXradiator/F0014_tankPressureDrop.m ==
function dp = F0014_tankPressureDrop(v, par)
% parameters
zeta = par.zeta;

% pressure drop
dp = 1/2 .* v .* abs(v) .* zeta;

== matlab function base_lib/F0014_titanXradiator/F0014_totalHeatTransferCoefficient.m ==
function U = F0014_totalHeatTransferCoefficient(v_air, v_clt, par)

% parameters
cU    = par.cU;
cUexp = par.cUexp;

% saturation
v_air = max(v_air, 0);
v_clt = max(v_clt, 0);


% Heat transfer coefficient
temp = cU(1) + cU(2) .* v_air.^-cUexp(1) + cU(3)*v_clt .^ -cUexp(2);
U    = 1./temp;

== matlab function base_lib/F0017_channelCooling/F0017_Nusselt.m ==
function Nu = F0017_Nusselt(Re, Pr, par)

% parameters
d = par.d;
L = par.L;

% Hausen Nusselt Correlation:
Nu_lam = 3.66 + ...
    (0.0668.*(d./L) .* Re .* Pr) ./ ...
    (1 + 0.04 .*( max( (d./L) .* Re .* Pr , 1e-10) ).^(2/3) );

% Sieder-Tate Correlation:
Nu_turb = 0.027 .* Re.^0.8 .* Pr.^(1/3);

% transition from laminar to turbulent flow
y = (Re-3500) / 2e3;
y = tanh(y*5)/2 + 1/2;

% Nusselt number
Nu = (1-y) .* Nu_lam + y.*Nu_turb;

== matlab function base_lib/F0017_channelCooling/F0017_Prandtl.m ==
function Pr = F0017_Prandtl(par)
% parameters
cp = par.cp_clt;
mu = par.mu_clt;
k  = par.k_clt;

% Prandtl number
Pr = cp .* mu ./ k;

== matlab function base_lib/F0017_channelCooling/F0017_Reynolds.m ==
function Re = F0017_Reynolds(v, par)
% parameters
rho = par.rho_clt;
mu  = par.mu_clt;
d   = par.d;

% Pipe reynolds number
Re = rho .* v .* d ./ mu;

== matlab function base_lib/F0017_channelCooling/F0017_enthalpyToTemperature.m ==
function T = F0017_enthalpyToTemperature(H, par)
    % parameters
    T0 = par.T0_clt;
    H0 = par.H0_clt;
    cp = par.cp_clt;
    
    % temperature
    T = T0 + 1./cp .* (H - H0);

end

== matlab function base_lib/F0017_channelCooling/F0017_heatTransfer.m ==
function [Q, T_2] = F0017_heatTransfer(T_1, T_w, Nu, W, par)
% Holman example 6-2, Heating of water in Laminar tube flow
% parameters
k  = par.k_clt;
cp = par.cp_clt;
d  = par.d;
L  = par.L;

% heat transfer coefficient
h = k .* Nu ./ d;

% factors
c1 =  W .* cp; 
c2 =  h.*pi.*d.*L;

% outlet temperature
T_2p = (c2 .* T_w + (c1 - c2./2) .* T_1 )./(c1 + c2./2);

% check if temperature reaches wall temperature
if T_1 < T_w
    % cooling
    T_2 = min(T_2p, T_w);
else
    % heating
    T_2 = max(T_2p, T_w);
end
    
% heat transfer
Q = W .* cp .* (T_2 - T_1);

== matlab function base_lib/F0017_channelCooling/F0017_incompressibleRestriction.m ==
function dp = F0017_incompressibleRestriction(W, dr,  par)

% parameters
C_d = par.C_d;
d   = par.d;
rho = par.rho_clt;

% restriction area
Ar = dr.^2 * pi / 4;

% diameter ratio
beta = dr./d;

% volumetric flow
Q = W ./ rho;

% pressure drop
dp = 1/2 .* rho .* (1 - beta.^4) .* (Q ./ (C_d .* Ar)).^2;

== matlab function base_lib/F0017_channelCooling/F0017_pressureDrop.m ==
function dp = F0017_pressureDrop(v, Re,  par)
% parameters
rho = par.rho_clt;
d   = par.d;
L   = par.L;
e   = par.e;

% Darcy-weisbach friction factor
% laminar
f_lam = 64 ./ (Re + 0.01);

% turbulent and roughness
kd     = e./d;
f_turb = 4./(-3.6 .* log10(6.9 ./ (Re+0.001) + (kd./3.7).^(10/9) )).^2;

% smooth transition between laminar & turbulent
y = (Re-2100) / 500;
y = tanh(y*5)/2 + 1/2;

% combined
f = y .* f_turb + (1-y).* f_lam;

% pressure drop
dp =  L .* f .* rho./2 .* v.^2 ./ d;

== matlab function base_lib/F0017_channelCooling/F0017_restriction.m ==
function dp = F0017_restriction(W, par)

% Discharge coefficient
C   = par.C;
d   = par.d;
rho = par.rho_clt; 

% Area
A = pi .* d.^2 / 4;

% Laminar restriction
dp = 1./rho .* (W ./ (C.*A));

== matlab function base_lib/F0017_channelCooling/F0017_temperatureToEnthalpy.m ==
function H = F0017_temperatureToEnthalpy(T, par)
    % parameters
    T0 = par.T0_clt;
    H0 = par.H0_clt;
    cp = par.cp_clt;
    
    % enthalpy
    H = H0 + cp.*(T - T0);

end

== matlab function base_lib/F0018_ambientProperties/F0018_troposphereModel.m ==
function [p,T] = F0018_troposphereModel(h, par)

% parameters
T_0 = par.T_0;
p_0 = par.p_0;

% The nasa troposphere model for pressure.
T = T_0 - 0.00649 .* h;
p = p_0 .* (T./288.078).^5.256;

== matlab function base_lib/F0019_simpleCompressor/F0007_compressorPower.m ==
function P_c = F0007_compressorPower(W_c, T_us, T_ds)

% model constants
g   = 1.4;
R   = 280;
cp  = g*R/(g-1);

% compressor work
P_c = cp .* W_c .* (T_ds - T_us);

end

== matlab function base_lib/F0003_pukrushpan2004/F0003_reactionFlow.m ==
function [W_an, W_ca] = F0003_reactionFlow(I)
% constants
F     = 96485; % [C/mol]  - Faradays constant
M_H2  = 0.002; % [kg/mol] - hydrogen molecular weight
M_O2  = 0.032; % [kg/mol] - oxygen   molecular weight
% M_N2  = 0.028; % [kg/mol] - nitrogen molecular weight
M_H2O = 0.018; % [kg/mol] - water    molecular weight

% reaction flows
W_H2_rct  = I * M_H2  /(2*F);
W_O2_rct  = I * M_O2  /(4*F);
W_H2O_rct = I * M_H2O /(2*F);

% output
W_an = [-W_H2_rct;         0;         0; 0];
W_ca = [        0; -W_O2_rct; W_H2O_rct; 0]; 
end

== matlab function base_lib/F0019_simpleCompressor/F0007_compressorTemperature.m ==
function T_ds = F0007_compressorTemperature(p_us, p_ds, T_us, eta_c)

% model constants
g = 1.4;

% pressure ratio
PiC = p_ds./p_us;

% compressor out temperature (adiabatic)
T_ds = T_us + T_us ./ eta_c .* ( PiC.^((g-1)/g)  - 1  );

end

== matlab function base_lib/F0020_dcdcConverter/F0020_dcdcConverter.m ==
function [eta, I_bus, P_bus, Q_gen] = F0020_dcdcConverter(U_bus, U_s, I, par)
% Function for the DC-DC converter connected to a DC-bus. The system
% connected to the converter can be either a consumer or a producer.
% Negative current, I, means that the connected device is a consumer from
% the DC-bus and a positive current means that the connected device is a
% producer to the DC-bus.


% Output:
% - eta: Voltage change efficiency
% - I_bus: Current to and from the DC Bus.
% - P_bus: Power to and from the DC Bus
% - P_loss: Converting loss, always positive.
% Inputs:
% - U_bus: DC Bus Voltage
% - U_s: System voltage connected to converter
% - I: Current to DC Bus (negative current is a consumer, positive a producer.)
% - eta_down: Buck Efficiency
% - eta_up: Boost Efficiency


% parameters
eta_down = par.eta_down;
eta_up   = par.eta_up;


producer = false;
U_out = 0;
U_in  = 0;

% producer/consumer mode:
if( I < 0 ) 
    % ... consumer from bus
    U_out = U_s;
    U_in  = U_bus;
else
    % ... producer to bus
    producer = true;
    U_out    = U_bus;
    U_in     = U_s;
end

% buck/boost mode:
if( U_out < U_in )
    % Buck conversion
    eta = eta_down;
else 
    % Boost conversion
    eta = eta_up;
end


P_s = U_s*I;

if( producer )
    P_bus = P_s*eta;
    I_bus = P_bus/U_bus;
else
    P_bus = P_s/eta;
    I_bus = P_bus/U_bus;
end

% heat generation
% P_bus < P_s < 0 for consumer current.
Q_gen = P_s-P_bus; 

end

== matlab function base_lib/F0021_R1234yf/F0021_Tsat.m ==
function Tsat = F0021_Tsat(p)

% critical properties
Tc   =     367.85; % [K]
pc   = 	3382200.0; % [Pa]
rhoc =     4170.0; % [mol/m3]

p = max(p,0);
p = min(p, pc);

% coefficients
x = [ 0.011785783765939;
  -0.000711388291699;
  -0.000000004534501;
   0.000005602194397;
   0.000000550569193 ];

% calculate saturated temperature
pr   = p ./ pc;
A    = [ones(size(p)), log(pr), log(pr).^2, log(pr).^3, log(pr).^4];
Tsat = exp( ( A * x ).^(-0.4) );

end

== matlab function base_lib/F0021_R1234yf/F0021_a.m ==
function a = F0021_a(T,rho)
%R1234yf_a
%    A = R1234yf_a(T,RHO)

%    This function was generated by the Symbolic Math Toolbox version 9.3.
%    16-Oct-2023 15:47:49

t2 = rho.^2;
t3 = rho.^3;
t4 = 1.0./T;
t5 = rho./4.17e+3;
t6 = -t5;
t8 = t4.*3.6785e+2;
t9 = t2./1.73889e+7;
t7 = exp(t6);
t10 = -t9;
t11 = t8.^(7.0./2.0);
t12 = exp(t10);
et1 = t4.*2.95847224925e+3+log(-exp(t4.*-7.18e+2)+1.0).*7.549+log(-exp(t4.*-8.77e+2)+1.0).*1.537+log(-exp(t4.*-1.755e+3)+1.0).*7.455+log(-exp(t4.*-4.465e+3)+1.0).*(2.03e+2./1.0e+2)+log(t5)+log(t8).*(6.18e+2./1.25e+2)+rho.*t8.^(8.0./2.5e+1).*3.709731414868106e-4;
et2 = rho.*t8.^(9.29e+2./1.0e+3).*(-5.64805035971223e-4)+t2.^2.*t4.*5.587038487243495e-14+t3.*t8.^(1.9e+1./5.0e+1).*2.424466237613225e-12;
et3 = t2.*t8.^(4.7e+1./5.0e+1).*(-2.776388960773827e-8)-rho.*t8.^(5.7e+1./2.5e+1).*t12.*2.901693045563549e-4-t3.*t8.^(4.4e+1./2.5e+1).*t12.*8.518739586251397e-12;
et4 = t2.*t8.^(6.1e+1./2.5e+1).*t12.*(-4.007473158164116e-8)+t2.*t7.*t8.^(9.7e+1./1.0e+2).*3.913566700596357e-8+t2.*t11.*exp((t8-6.0./5.0).^2.*-1.08e+2-(t5-4.1e+1./2.5e+1).^2.*(8.1e+1./5.0)).*1.971683660266032e-11;
et5 = t3.*t4.*exp((t8-3.2e+1./2.5e+1).^2.*-8.0e+1-(t5-3.59e+2./5.0e+2).^2.*(1.46e+2./2.5e+1)).*(-5.821977769301905e-9)-t3.*t11.*exp((t8-2.3e+1./5.0e+1).^2.*(-8.9e+1./1.0e+2)-(t5-6.77e+2./1.0e+3).^2.*(2.11e+2./2.0e+2)).*2.723951646267135e-12;
et6 = rho.^7.*t7.*t8.^(2.1e+1./2.0e+1).*(-1.229509534838242e-27)+rho.*t8.^(7.0./5.0).*exp((t5-8.9e+1./1.25e+2).^2.*(-5.1e+1./5.0e+1)-(t8-1.13e+2./1.0e+2).^2.*(7.1e+1./5.0e+1)).*3.333251798561151e-4;
et7 = rho.*t4.^3.*exp((t8-6.7e+1./1.0e+2).^2.*(-2.31e+2./1.0e+2)-(t5-9.1e+1./1.0e+2).^2.*(1.67e+2./1.25e+2)).*(-5.702218194789895e+3)-1.2837928e+1;
a = T.*(et1+et2+et3+et4+et5+et6+et7).*8.314472;
end
